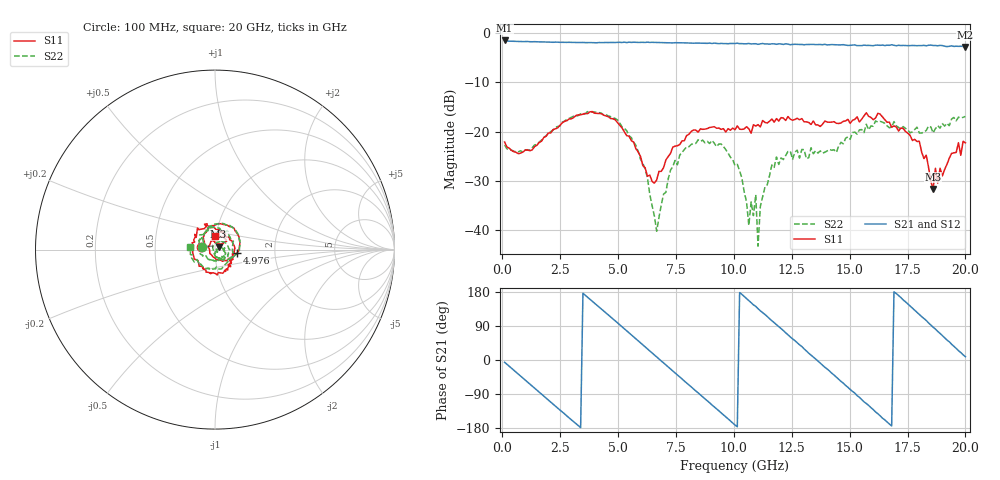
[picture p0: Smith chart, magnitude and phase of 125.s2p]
!Agilent Technologies,N5230C,MY49001569,A.09.33.09
!Agilent N5230C: A.09.33.09
!Date: Monday, July 27, 2015 15:29:57
!Correction: S11(Full 2 Port(1,2))
!S21(Full 2 Port(1,2))
!S12(Full 2 Port(1,2))
!S22(Full 2 Port(1,2))
!S2P File: Measurements: S11, S21, S12, S22:
# Hz S  dB  R 50
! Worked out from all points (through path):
!   201 points, 100 MHz to 20 GHz, reference 50 ohm
!   highest |S21| = -1.56 dB at 100 MHz (marker M1); lowest = -2.8 dB at 20 GHz (marker M2)
!   group delay of S21, straight-line fit = 148 ps
!   lowest |S11| = -31.6 dB at 18.61 GHz (marker M3), VSWR 1.05, Z = 52 + j1.74 ohm
!   |S11| at or under -10 dB: start of sweep to end of sweep
!   |S22| runs from -43.2 to -16.0 dB; largest |S21 - S12| = 0.032
!   S11 on the Smith chart (normalised r, x): 100 MHz: 0.86, +0.02; 4.976 GHz: 1.28, -0.05; 20 GHz: 0.99, +0.15
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1e8  -22.13 170.5  -1.56 -6.0  -1.62 -5.8  -22.72 169.6
1.7915e9  -21.21 137.7  -1.87 -95.3  -1.86 -95.2  -21.22 141.2
3.483e9  -16.49 66.7  -1.96 176.1  -1.98 175.9  -16.33 70.7
4.9755e9  -18.19 -8.7  -1.95 98.1  -1.96 97.8  -17.65 -9.4
5.7715e9  -23.52 -61.6  -1.93 55.8  -1.96 55.5  -22.82 -52.1
6.667e9  -29.83 173.0  -1.94 8.2  -1.94 7.9  -40.19 -166.4
6.7665e9  -28.07 159.5  -1.97 2.7  -1.98 2.7  -37.38 153.3
7.463e9  -22.96 89.1  -2.01 -34.2  -2.02 -34.2  -25.86 58.7
8.458e9  -20.12 34.2  -2.10 -86.7  -2.10 -87.3  -21.69 0.3
1.005e10  -19.64 -23.7  -2.17 -171.6  -2.25 -171.4  -26.90 -71.7
1.0647e10  -19.45 -36.8  -2.16 156.7  -2.22 156.3  -39.01 -78.2
1.09455e10  -18.88 -43.2  -2.22 141.7  -2.21 140.3  -32.81 -48.2
1.1045e10  -18.61 -40.2  -2.34 135.4  -2.28 135.4  -43.22 17.3
1.11445e10  -19.06 -49.4  -2.24 129.8  -2.25 130.4  -35.14 3.1
1.1841e10  -17.38 -64.4  -2.34 93.5  -2.39 92.7  -25.15 10.2
1.3433e10  -17.87 -133.7  -2.35 8.3  -2.45 8.0  -24.51 -79.8
1.5025e10  -18.35 159.7  -2.54 -77.7  -2.46 -78.5  -21.58 176.7
1.5821e10  -16.91 129.1  -2.55 -119.8  -2.63 -120.8  -19.66 126.1
1.67165e10  -18.10 92.5  -2.54 -169.0  -2.53 -169.4  -19.24 67.2
1.801e10  -21.97 35.3  -2.59 120.1  -2.64 119.4  -20.28 -26.1
1.8607e10  -31.65 39.6  -2.57 86.6  -2.69 86.1  -20.29 -85.6
2e10  -22.29 90.8  -2.85 8.7  -2.81 7.7  -16.94 173.6
